{attribute 'qualified_only'}
VAR_GLOBAL CONSTANT
	CamTablePoints											: INT		:= 10;		// 凸轮表点位个数 
	MIN_SLAVES												: 	UINT  := 1;
	MAX_SLAVES												: 	UINT  := 1000;
	MIN_ANALOGVALUE											:	LREAL := 0;
	MAX_ANALOGVALUE											:	LREAL := 32767;
	TimeZone                 							    :   INT   := 30;			// FB_SignalAlarmRecord
	MaxReadSizeBuff											: UDINT		:= 1024;
END_VAR
